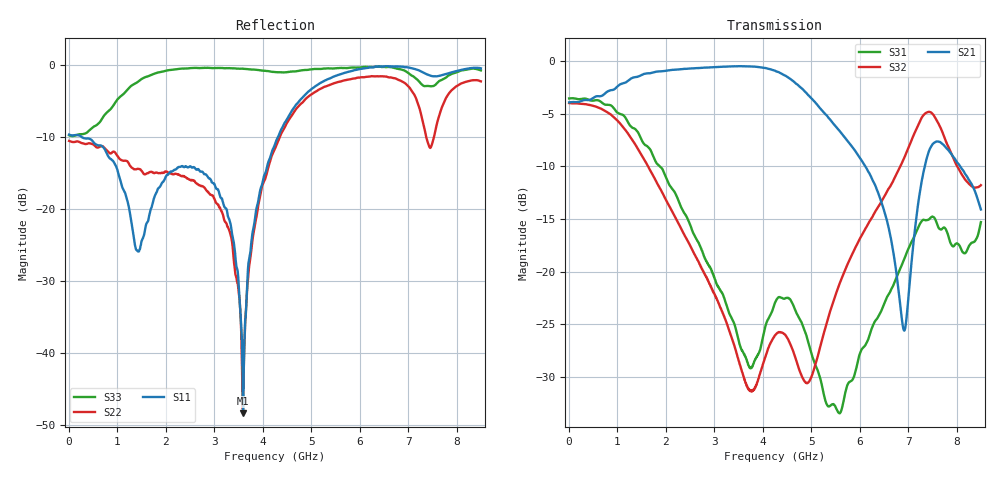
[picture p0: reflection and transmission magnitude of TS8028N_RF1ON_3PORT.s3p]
!Created with skrf (http://scikit-rf.org).
# GHz S RI R 50.0
!freq ReS11 ImS11 ReS12 ImS12 ReS13 ImS13
! ReS21 ImS21 ReS22 ImS22 ReS23 ImS23
! ReS31 ImS31 ReS32 ImS32 ReS33 ImS33
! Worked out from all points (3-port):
!   1601 points, 10 MHz to 8.5 GHz, reference 50 ohm
!   strongest paths, dB at 10 MHz, 2.132 GHz, 4.255 GHz, 6.378 GHz, 8.5 GHz:
!     S21: -3.9, -0.8, -0.9, -12.4, -14.1
!     S32: -4.0, -14.3, -26.0, -13.9, -11.8
!     S31: -3.5, -12.1, -23.0, -24.3, -15.3
!   lowest |S11| = -48.4 dB at 3.597 GHz (marker M1), VSWR 1.01, Z = 50.3 + j0.186 ohm
!   |S11| at or under -10 dB: 276.8 MHz to 4.316 GHz (4.039 GHz wide, 176 % of centre)
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0.01  -0.3303 0.00676  0.6376 0.00211  0.6657 -0.00456
      0.6373 0.00204  -0.2985 0.00726  0.6323 -0.00607
      0.6655 -0.00472  0.6325 -0.006  -0.3268 0.0139
1.564731  0.068 0.0111  0.7953 -0.3573  -0.0734 -0.3957
          0.7951 -0.3575  -0.123 0.1244  -0.111 -0.3211
          -0.0734 -0.3953  -0.111 -0.3214  0.8005 -0.1986
2.960275  0.1251 -0.0883  0.3826 -0.8533  -0.0868 -0.0491
          0.3823 -0.8536  0.00306 0.1243  -0.0797 -0.0218
          -0.0868 -0.0489  -0.0795 -0.0218  0.2578 -0.9236
3.597025  0.00332 0.00185  0.0507 -0.9456  -0.0324 -0.0258
          0.0503 -0.9454  -0.0046 0.000207  -0.0226 0.0228
          -0.0325 -0.0258  -0.0226 0.0228  -0.26 -0.9123
4.255  -0.0253 0.2819  -0.3694 -0.823  -0.0304 -0.0645
       -0.3706 -0.8217  -0.2112 -0.1588  0.049 -0.00857
       -0.0306 -0.0643  0.0491 -0.0085  -0.8997 -0.00133
4.7644  0.0682 0.5657  -0.5603 -0.5089  -0.0587 -0.0101
        -0.5613 -0.5076  -0.5318 -0.00988  0.0243 -0.0234
        -0.0586 -0.00991  0.0242 -0.0234  -0.1901 0.8993
5.767281  0.0952 0.8983  -0.4084 -0.0671  0.0239 0.0174
          -0.4082 -0.0666  -0.2968 0.7412  0.1091 -0.0182
          0.0239 0.0174  0.1092 -0.0181  0.6299 0.7263
6.918737  0.192 0.9549  -0.0376 -0.0368  0.0916 -0.0693
          -0.0376 -0.0366  0.6095 0.4512  0.1884 -0.2903
          0.0912 -0.0696  0.1898 -0.2907  0.7227 0.5766
7.369769  0.1094 0.8662  -0.0793 -0.3272  0.0156 -0.1752
          -0.0792 -0.3273  0.1181 -0.2988  -0.1663 -0.5445
          0.0162 -0.1749  -0.1659 -0.5438  0.4511 0.5603
8.5  -0.4345 0.8504  -0.1958 -0.0287  -0.1719 0.004
     -0.1955 -0.0286  0.5833 0.5102  -0.2048 0.1562
     -0.1719 0.00392  -0.205 0.1562  0.3412 0.8586
